(* Logix 5000 AddOnInstructionDefinition export Banner_LCA_PD_v4; software revision 33.00 *)

TYPE Banner_LCA_Adv_v4 :   // Advanced Process Data information for a Banner LCA.
STRUCT
   Type : SINT;   // 0 = Off, 1 = Steady, 2 = Flash, 3= Two Color Flash, 4 = Intensity Sweep, 5 = Color Sweep.
   Output : SINT;   // 0 = Off, 1 = On, 2 = Pattern.
   Pattern : SINT;   // 0 = Flash, 1 = Strobe, 2 = Three Pulse, 3 = SOS, 4 = Random.
   Speed : SINT;   // 0 = Slow, 1 = Medium, 2 = Fast, 3 = Custom.
   Color_1 : SINT;   // 0 = Green, 1 = Red, 2 = Orange, 3 = Amber, 4 = Yellow, 5 = Lime Green, 6 = Spring Green, 7 = Cyan, 8 = Sky Blue, 9 = Blue, 10 = Violet, 11 = Magenta, 12 = Rose, 13 = White, 14 = Custom 1, 15 = Custom 2.
   Color_1_Intensity : SINT;   // 0 = High, 1 = Medium, 2 = Low, 3 = Off, 4 = Custom.
   Color_2 : SINT;   // 0 = Green, 1 = Red, 2 = Orange, 3 = Amber, 4 = Yellow, 5 = Lime Green, 6 = Spring Green, 7 = Cyan, 8 = Sky Blue, 9 = Blue, 10 = Violet, 11 = Magenta, 12 = Rose, 13 = White, 14 = Custom 1, 15 = Custom 2.
   Color_2_Intensity : SINT;   // 0 = High, 1 = Medium, 2 = Low, 3 = Off, 4 = Custom.
END_STRUCT
END_TYPE

TYPE Banner_LCA_Advanced_v4 :   // Advanced Process Data.
STRUCT
   Output_Status : SINT[6];   // 0 = Off, 1= On.
   Button : Banner_LCA_Adv_v4[6];
END_STRUCT
END_TYPE

TYPE Banner_LCA_PDIO_v4 :   // UDT that records the converted prcoess data.
STRUCT
   State : Banner_LCA_State_v4;   // Only active when Operation Mode set to 0. State tells the light which of the four states it should be in. 0 = State 1, 1 = State 2, 2 = State 3, 3 = State 4.
   Advanced : Banner_LCA_Advanced_v4;   // Only active when Operation Mode set to 2.
   DTO : SINT[20];
   DTI : SINT[2];
END_STRUCT
END_TYPE

TYPE Banner_LCA_State_v4 :
STRUCT
   Output_Status : SINT[6];   // 0 = Reserved, 1 = Off, 2 = On, 3 = Hold. Current status of Output.
   Output_State : SINT[6];   // 0 = No Overide, 1 Off, 2 = On, 3 = Hold. Related parameters defined in outptu and touch settings parameter data.
END_STRUCT
END_TYPE

ADD_ON_INSTRUCTION Banner_LCA_PD_v4   (* revision 4.0, vendor Banner Engineering *)
// Takes the raw SINT information and converts that data into actual information.
VAR_IN_OUT
   PD : Banner_LCA_PDIO_v4; {required}
END_VAR
VAR_INPUT
   Mode : SINT; {required}   // Linked from Parameters AOI or entered manually.
   Byte_Swap : BOOL; {required}
END_VAR
VAR
   PDO_Temp : SINT[20]; {access None}
   PDI_Temp : SINT[2]; {access None}
END_VAR

ROUTINE Logic   (* ladder *)
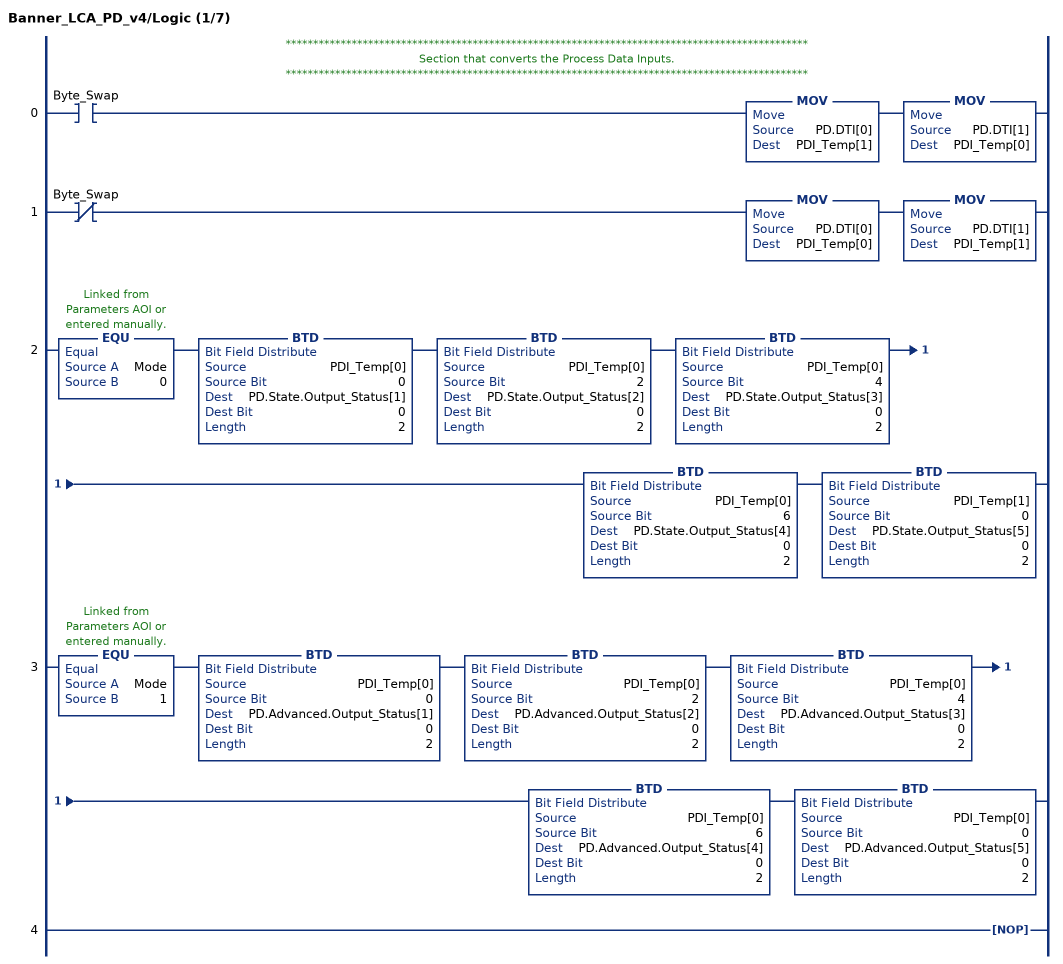
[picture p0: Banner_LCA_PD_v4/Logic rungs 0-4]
   // ***********************************************************************************************
   // Section that converts the Process Data Inputs.
   // ***********************************************************************************************
   0: XIC(Byte_Swap)MOV(PD.DTI[0],PDI_Temp[1])MOV(PD.DTI[1],PDI_Temp[0]);
   1: XIO(Byte_Swap)MOV(PD.DTI[0],PDI_Temp[0])MOV(PD.DTI[1],PDI_Temp[1]);
   2: EQU(Mode,0)BTD(PDI_Temp[0],0,PD.State.Output_Status[1],0,2)BTD(PDI_Temp[0],2,PD.State.Output_Status[2],0,2)BTD(PDI_Temp[0],4,PD.State.Output_Status[3],0,2)BTD(PDI_Temp[0],6,PD.State.Output_Status[4],0,2)BTD(PDI_Temp[1],0,PD.State.Output_Status[5],0,2);
   3: EQU(Mode,1)BTD(PDI_Temp[0],0,PD.Advanced.Output_Status[1],0,2)BTD(PDI_Temp[0],2,PD.Advanced.Output_Status[2],0,2)BTD(PDI_Temp[0],4,PD.Advanced.Output_Status[3],0,2)BTD(PDI_Temp[0],6,PD.Advanced.Output_Status[4],0,2)BTD(PDI_Temp[0],0,PD.Advanced.Output_Status[5],0,2);
   4: NOP();
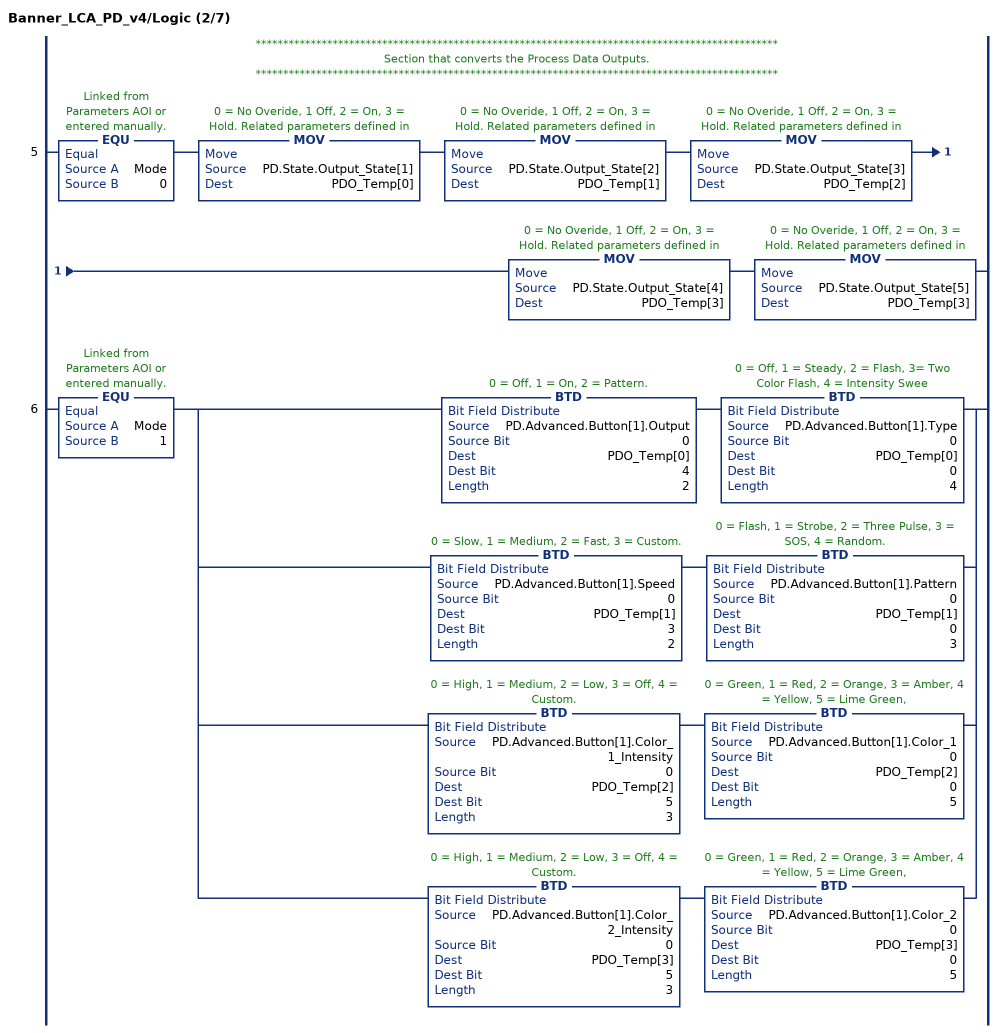
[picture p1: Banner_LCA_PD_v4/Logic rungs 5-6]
   // ***********************************************************************************************
   // Section that converts the Process Data Outputs.
   // ***********************************************************************************************
   5: EQU(Mode,0)MOV(PD.State.Output_State[1],PDO_Temp[0])MOV(PD.State.Output_State[2],PDO_Temp[1])MOV(PD.State.Output_State[3],PDO_Temp[2])MOV(PD.State.Output_State[4],PDO_Temp[3])MOV(PD.State.Output_State[5],PDO_Temp[3]);
   6: EQU(Mode,1)[BTD(PD.Advanced.Button[1].Output,0,PDO_Temp[0],4,2) BTD(PD.Advanced.Button[1].Type,0,PDO_Temp[0],0,4) ,BTD(PD.Advanced.Button[1].Speed,0,PDO_Temp[1],3,2) BTD(PD.Advanced.Button[1].Pattern,0,PDO_Temp[1],0,3) ,BTD(PD.Advanced.Button[1].Color_1_Intensity,0,PDO_Temp[2],5,3) BTD(PD.Advanced.Button[1].Color_1,0,PDO_Temp[2],0,5) ,BTD(PD.Advanced.Button[1].Color_2_Intensity,0,PDO_Temp[3],5,3) BTD(PD.Advanced.Button[1].Color_2,0,PDO_Temp[3],0,5) ];
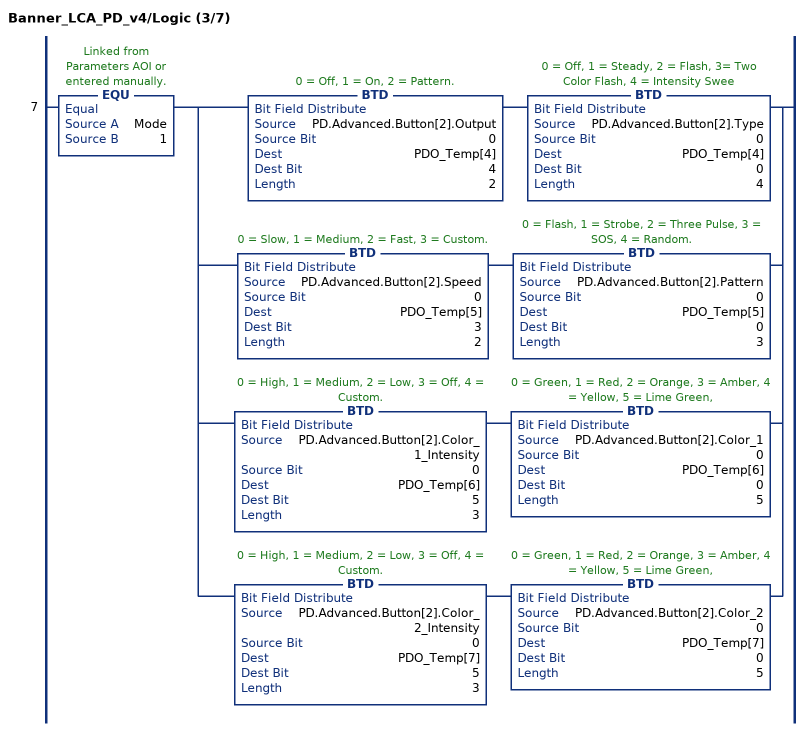
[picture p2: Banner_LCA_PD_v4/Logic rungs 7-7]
   7: EQU(Mode,1)[BTD(PD.Advanced.Button[2].Output,0,PDO_Temp[4],4,2) BTD(PD.Advanced.Button[2].Type,0,PDO_Temp[4],0,4) ,BTD(PD.Advanced.Button[2].Speed,0,PDO_Temp[5],3,2) BTD(PD.Advanced.Button[2].Pattern,0,PDO_Temp[5],0,3) ,BTD(PD.Advanced.Button[2].Color_1_Intensity,0,PDO_Temp[6],5,3) BTD(PD.Advanced.Button[2].Color_1,0,PDO_Temp[6],0,5) ,BTD(PD.Advanced.Button[2].Color_2_Intensity,0,PDO_Temp[7],5,3) BTD(PD.Advanced.Button[2].Color_2,0,PDO_Temp[7],0,5) ];
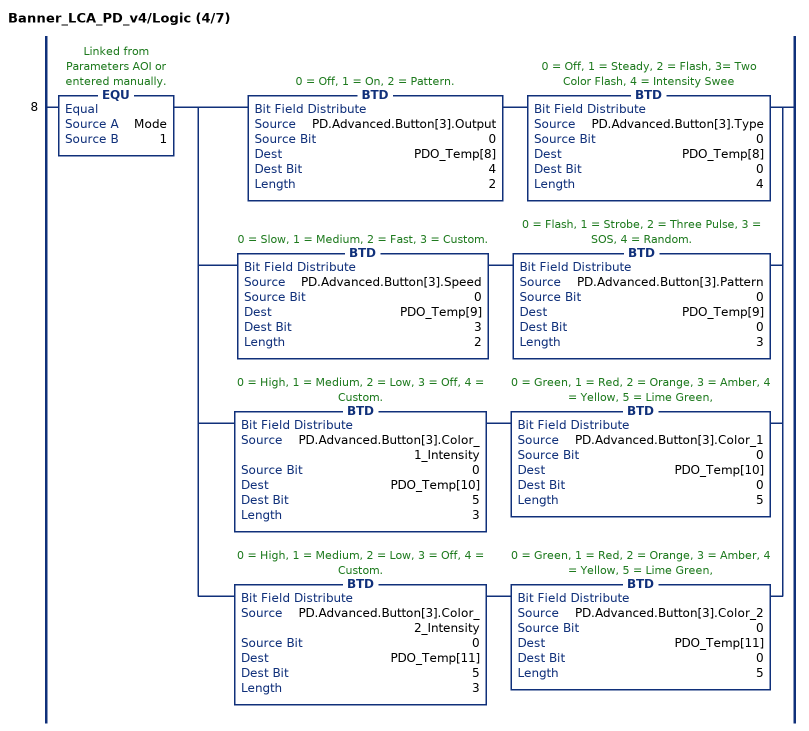
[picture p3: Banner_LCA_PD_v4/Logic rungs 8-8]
   8: EQU(Mode,1)[BTD(PD.Advanced.Button[3].Output,0,PDO_Temp[8],4,2) BTD(PD.Advanced.Button[3].Type,0,PDO_Temp[8],0,4) ,BTD(PD.Advanced.Button[3].Speed,0,PDO_Temp[9],3,2) BTD(PD.Advanced.Button[3].Pattern,0,PDO_Temp[9],0,3) ,BTD(PD.Advanced.Button[3].Color_1_Intensity,0,PDO_Temp[10],5,3) BTD(PD.Advanced.Button[3].Color_1,0,PDO_Temp[10],0,5) ,BTD(PD.Advanced.Button[3].Color_2_Intensity,0,PDO_Temp[11],5,3) BTD(PD.Advanced.Button[3].Color_2,0,PDO_Temp[11],0,5) ];
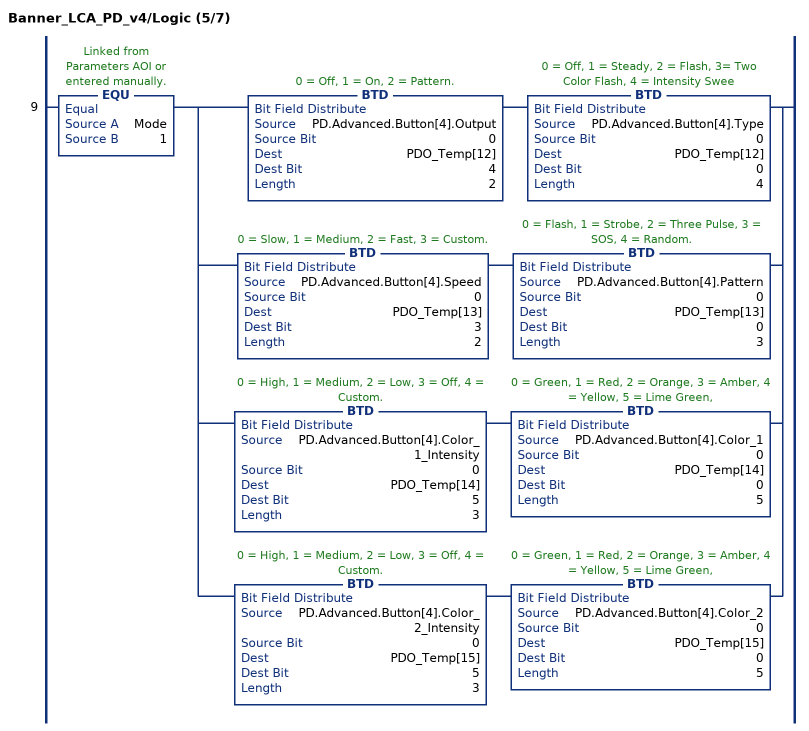
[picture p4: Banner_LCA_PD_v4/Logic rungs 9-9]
   9: EQU(Mode,1)[BTD(PD.Advanced.Button[4].Output,0,PDO_Temp[12],4,2) BTD(PD.Advanced.Button[4].Type,0,PDO_Temp[12],0,4) ,BTD(PD.Advanced.Button[4].Speed,0,PDO_Temp[13],3,2) BTD(PD.Advanced.Button[4].Pattern,0,PDO_Temp[13],0,3) ,BTD(PD.Advanced.Button[4].Color_1_Intensity,0,PDO_Temp[14],5,3) BTD(PD.Advanced.Button[4].Color_1,0,PDO_Temp[14],0,5) ,BTD(PD.Advanced.Button[4].Color_2_Intensity,0,PDO_Temp[15],5,3) BTD(PD.Advanced.Button[4].Color_2,0,PDO_Temp[15],0,5) ];
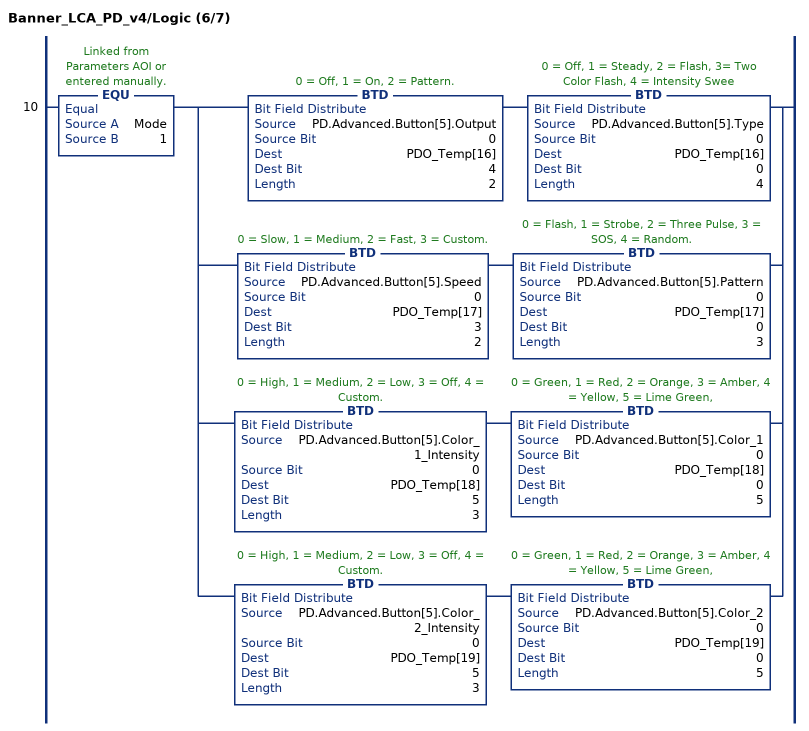
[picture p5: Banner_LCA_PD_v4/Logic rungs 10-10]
   10: EQU(Mode,1)[BTD(PD.Advanced.Button[5].Output,0,PDO_Temp[16],4,2) BTD(PD.Advanced.Button[5].Type,0,PDO_Temp[16],0,4) ,BTD(PD.Advanced.Button[5].Speed,0,PDO_Temp[17],3,2) BTD(PD.Advanced.Button[5].Pattern,0,PDO_Temp[17],0,3) ,BTD(PD.Advanced.Button[5].Color_1_Intensity,0,PDO_Temp[18],5,3) BTD(PD.Advanced.Button[5].Color_1,0,PDO_Temp[18],0,5) ,BTD(PD.Advanced.Button[5].Color_2_Intensity,0,PDO_Temp[19],5,3) BTD(PD.Advanced.Button[5].Color_2,0,PDO_Temp[19],0,5) ];
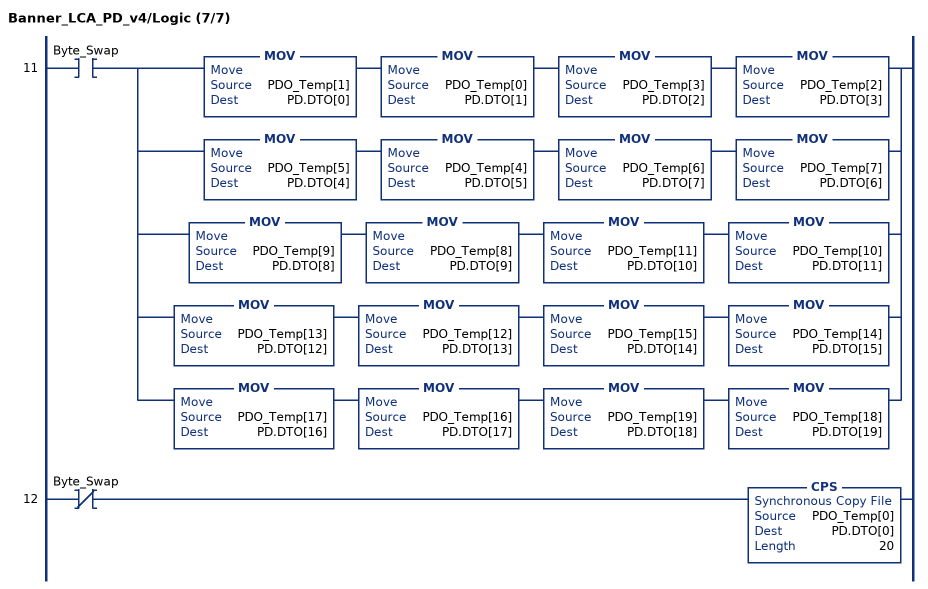
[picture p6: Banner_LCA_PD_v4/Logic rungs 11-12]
   11: XIC(Byte_Swap)[MOV(PDO_Temp[1],PD.DTO[0]) MOV(PDO_Temp[0],PD.DTO[1]) MOV(PDO_Temp[3],PD.DTO[2]) MOV(PDO_Temp[2],PD.DTO[3]) ,MOV(PDO_Temp[5],PD.DTO[4]) MOV(PDO_Temp[4],PD.DTO[5]) MOV(PDO_Temp[6],PD.DTO[7]) MOV(PDO_Temp[7],PD.DTO[6]) ,MOV(PDO_Temp[9],PD.DTO[8]) MOV(PDO_Temp[8],PD.DTO[9]) MOV(PDO_Temp[11],PD.DTO[10]) MOV(PDO_Temp[10],PD.DTO[11]) ,MOV(PDO_Temp[13],PD.DTO[12]) MOV(PDO_Temp[12],PD.DTO[13]) MOV(PDO_Temp[15],PD.DTO[14]) MOV(PDO_Temp[14],PD.DTO[15]) ,MOV(PDO_Temp[17],PD.DTO[16]) MOV(PDO_Temp[16],PD.DTO[17]) MOV(PDO_Temp[19],PD.DTO[18]) MOV(PDO_Temp[18],PD.DTO[19]) ];
   12: XIO(Byte_Swap)CPS(PDO_Temp[0],PD.DTO[0],20);
END_ROUTINE
END_ADD_ON_INSTRUCTION
